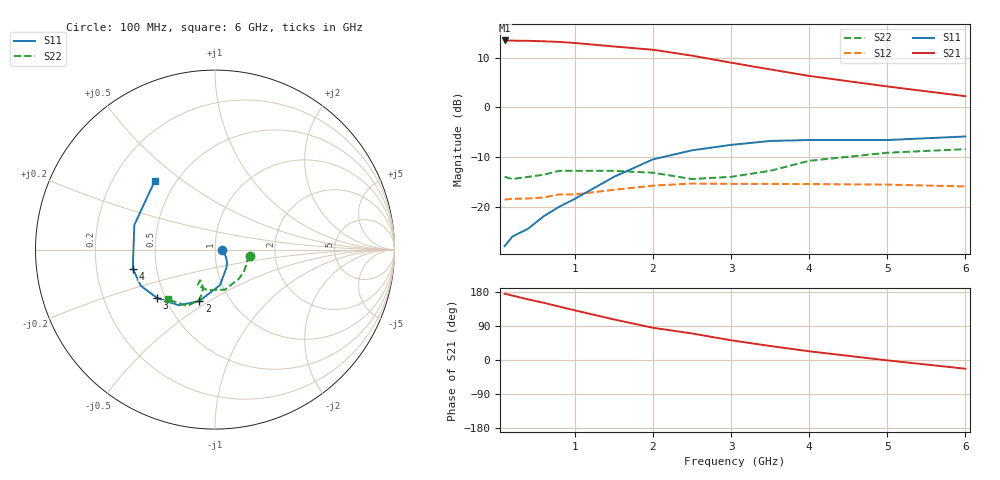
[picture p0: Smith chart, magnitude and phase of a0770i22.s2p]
!  MSA-0770 S AND NOISE PARAMETERS
!  Id=22mA  LAST UPDATED 07-27-92
# ghz s ma r 50
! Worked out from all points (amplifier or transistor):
!   14 points, 100 MHz to 6 GHz, reference 50 ohm
!   highest |S21| = 13.5 dB at 100 MHz (marker M1)
!   |S21| within 3 dB of that: start of sweep to 2.472 GHz
!   unconditionally stable (mu >= 1): start of sweep to 1.713 GHz; 2.879 GHz to end of sweep
!   at 400 MHz: K = 1.13, MAG = 13.7 dB, |S12| = -18.3 dB
!   at 2 GHz: K = 0.96, MSG = 13.7 dB, |S12| = -15.8 dB
!   at 6 GHz: K = 1.46, MAG = 5.1 dB, |S12| = -15.9 dB
!   lowest NFmin = 4.30 dB at 100 MHz
!   S11 on the Smith chart (normalised r, x): 100 MHz: 1.08, -0.01; 2 GHz: 0.72, -0.45; 3 GHz: 0.45, -0.30; 4 GHz: 0.36, -0.10; 6 GHz: 0.38, +0.40
0.1  0.04 -7.0  4.74 175.0  0.118 2.0  0.2 -10.0
0.2  0.05 -11.0  4.72 170.0  0.12 2.0  0.19 -18.0
0.4  0.06 -24.0  4.7 160.0  0.121 6.0  0.2 -34.0
0.6  0.08 -38.0  4.65 151.0  0.124 7.0  0.21 -50.0
0.8  0.1 -48.0  4.58 141.0  0.133 9.0  0.23 -76.0
1  0.12 -58.0  4.47 131.0  0.133 9.0  0.23 -76.0
1.5  0.2 -82.0  4.12 107.0  0.148 10.0  0.23 -101.0
2  0.3 -107.0  3.82 85.0  0.163 8.0  0.22 -116.0
2.5  0.37 -123.0  3.33 70.0  0.171 7.0  0.19 -116.0
3  0.42 -140.0  2.83 52.0  0.17 3.0  0.2 -111.0
3.5  0.46 -154.0  2.42 37.0  0.17 1.0  0.23 -107.0
4  0.47 -167.0  2.08 23.0  0.169 -4.0  0.29 -107.0
5  0.47 163.0  1.63 -1.0  0.167 -9.0  0.35 -116.0
6  0.51 131.0  1.3 -23.0  0.16 -11.0  0.38 -133.0
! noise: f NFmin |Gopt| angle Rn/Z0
0.1  4.3  0.05  5  0.6
0.5  4.4  0.06  26  0.59
1  4.5  0.06  55  0.58
2  5  0.06  116  0.56
